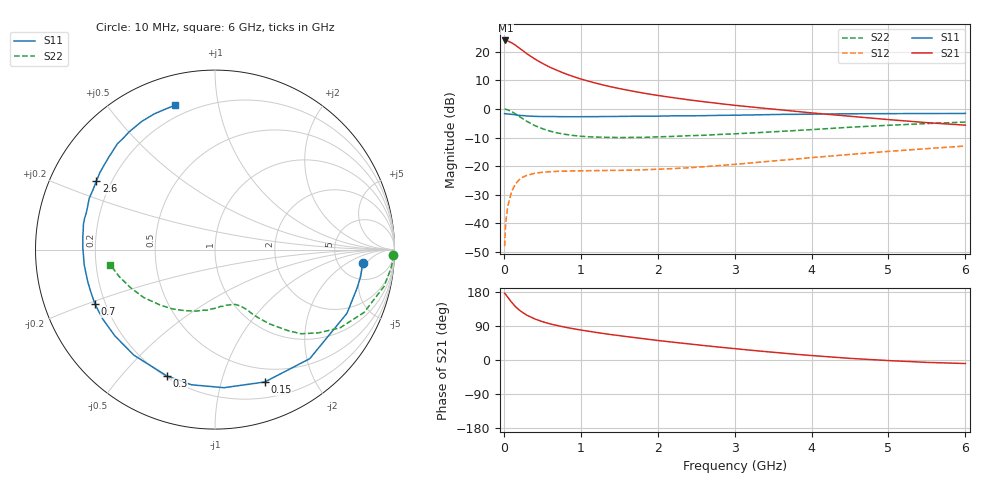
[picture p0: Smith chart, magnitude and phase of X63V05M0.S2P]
! SIEMENS Small Signal Semiconductors
! BFP193W
! Si NPN RF Bipolar Junction Transistor in SOT343
! VCE = 3 V  IC = 5 mA
! Common Emitter S-Parameters:  April 1994
# GHz  S  MA  R  50
!  f  S11  S21  S12  S22
! GHz  MAG  ANG  MAG  ANG  MAG  ANG  MAG  ANG
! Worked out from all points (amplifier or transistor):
!   40 points, 10 MHz to 6 GHz, reference 50 ohm
!   highest |S21| = 23.9 dB at 20 MHz (marker M1)
!   |S21| within 3 dB of that: start of sweep to 218.4 MHz
!   unconditionally stable (mu >= 1): 1.696 GHz to 4.36 GHz
!   at 200 MHz: K = 0.14, MSG = 23.0 dB, |S12| = -24.7 dB
!   at 1.5 GHz: K = 0.93, MSG = 14.3 dB, |S12| = -21.5 dB
!   at 6 GHz: K = 0.93, MSG = 3.6 dB, |S12| = -13.0 dB
!   lowest NFmin = 1.20 dB at 450 MHz
!   S11 on the Smith chart (normalised r, x): 10 MHz: 8.61, -3.97; 150 MHz: 0.36, -1.38; 300 MHz: 0.21, -0.67; 700 MHz: 0.16, -0.21; 2.6 GHz: 0.14, +0.26; 6 GHz: 0.14, +0.75
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0.01  0.8255 -5.1  15.64 176.3  0.004 87.4  0.9943 -1.7
0.02  0.8255 -10.4  15.71 174.2  0.0082 83.9  0.9886 -5.1
0.05  0.8163 -25.8  15.38 165.7  0.0195 76.7  0.9643 -12.2
0.1  0.805 -49.0  14.34 152.7  0.0359 65.7  0.9017 -22.8
0.15  0.788 -69.4  13.02 141.1  0.0487 55.8  0.8221 -32.0
0.2  0.771 -86.3  11.6 131.9  0.058 48.4  0.7403 -38.8
0.25  0.7645 -99.9  10.36 124.5  0.0646 42.3  0.6703 -44.4
0.3  0.7531 -110.9  9.205 118.2  0.0691 37.7  0.6058 -48.1
0.4  0.7419 -127.5  7.499 108.6  0.0749 31.2  0.5139 -53.7
0.5  0.7364 -139.2  6.266 101.2  0.0783 27.3  0.4527 -57.4
0.6  0.7355 -148.3  5.345 95.4  0.08 24.6  0.409 -60.2
0.7  0.7344 -155.5  4.68 90.7  0.0812 23.1  0.3792 -62.0
0.9  0.7311 -165.7  3.691 82.6  0.0827 21.6  0.3441 -65.9
1.1  0.7337 -173.6  3.061 75.9  0.0834 21.2  0.3259 -69.6
1.3  0.7364 179.6  2.6 69.8  0.0839 21.9  0.3196 -73.7
1.6  0.7423 171.5  2.138 61.6  0.0852 24.3  0.3171 -79.7
2.2  0.7567 157.9  1.573 47.0  0.0907 30.4  0.3308 -93.1
2.6  0.763 150.1  1.336 38.2  0.0978 34.9  0.3462 -102.4
3.2  0.7839 139.2  1.088 26.0  0.1134 39.5  0.3789 -116.1
4.5  0.8225 119.9  0.745 4.3  0.1603 41.5  0.4788 -146.1
5.5  0.8297 109.9  0.576 -6.3  0.2024 38.0  0.555 -164.4
6  0.835 105.3  0.52 -9.3  0.2249 35.7  0.5888 -171.7
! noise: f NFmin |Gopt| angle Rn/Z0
0.45  1.2  0.26  102  0.14
0.9  1.25  0.38  145  0.12
1.8  2.05  0.56  -161  0.12
